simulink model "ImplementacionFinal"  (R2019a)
settings: Solver=FixedStepAuto  StartTime=0.0  StopTime=Inf  RelTol=1e-3  EnableMultiTasking=on
undefined symbols (not defined in the file): ADCIN0, ADCIN1, ADCINA0, ADCINB0, bit, ended, input, Single
libraries: c2837xDlib x6, powerlib_meascontrol x5, simulink x4, c2802xlib x3

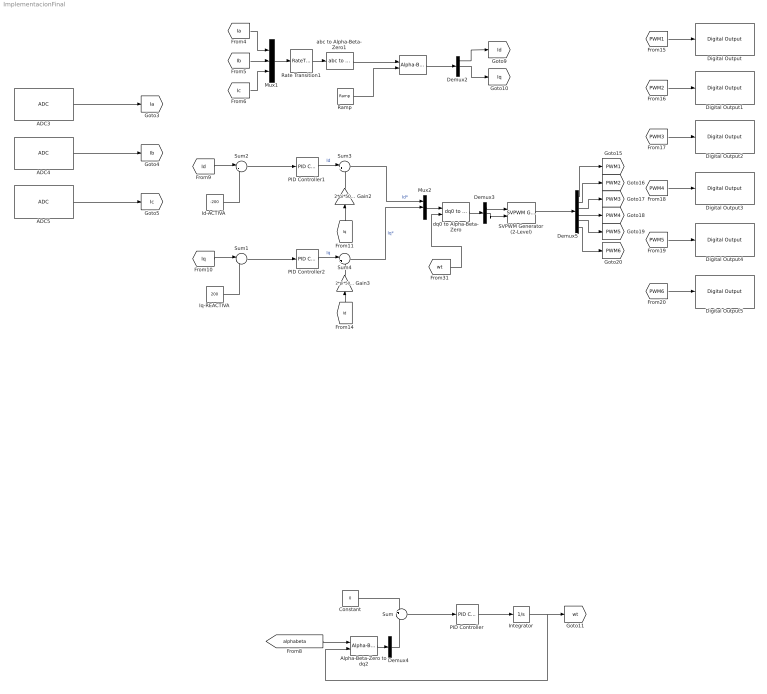
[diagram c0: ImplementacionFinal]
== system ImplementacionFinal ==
  " " : powerlib_meascontrol/Transformations/Alpha-Beta-Zero to dq0  Alignment=90 degrees behind phase A axis
  ADC3 : c2802xlib/ADC  blkParamProc=C2000_Type4  ADCModule=C  samplingMode=Single sample mode  ADCResolution=12-bit (Single-ended input)  useSOC1=SOC0  useSOC2=SOC0_SOC1  SOCAcquisitionWindow=15  SOCTriggerSource=Software  SOCInterruptTrigger=No ADCINT  Ts=0.001  dType=double  postInterrupt=off  interruptSel=ADCINT1  ADCINTContinuous=on  endma=off  chdma=1  conv1=ADCINA0  conv2=ADCINA0 and ADCINB0  conv1_Type4=ADCIN2  conv2_Type4=ADCIN0 and ADCIN1
  ADC4 : c2802xlib/ADC  blkParamProc=C2000_Type4  ADCModule=B  samplingMode=Single sample mode  ADCResolution=12-bit (Single-ended input)  useSOC1=SOC1  useSOC2=SOC0_SOC1  SOCAcquisitionWindow=15  SOCTriggerSource=Software  SOCInterruptTrigger=No ADCINT  Ts=0.001  dType=double  postInterrupt=off  interruptSel=ADCINT1  ADCINTContinuous=on  endma=off  chdma=1  conv1=ADCINA0  conv2=ADCINA0 and ADCINB0  conv1_Type4=ADCIN2  conv2_Type4=ADCIN0 and ADCIN1
  ADC5 : c2802xlib/ADC  blkParamProc=C2000_Type4  ADCModule=A  samplingMode=Single sample mode  ADCResolution=12-bit (Single-ended input)  useSOC1=SOC2  useSOC2=SOC0_SOC1  SOCAcquisitionWindow=15  SOCTriggerSource=Software  SOCInterruptTrigger=No ADCINT  Ts=0.001  dType=double  postInterrupt=off  interruptSel=ADCINT1  ADCINTContinuous=on  endma=off  chdma=1  conv1=ADCINA0  conv2=ADCINA0 and ADCINB0  conv1_Type4=ADCIN2  conv2_Type4=ADCIN0 and ADCIN1
  Alpha-Beta-Zero to dq2 : powerlib_meascontrol/Transformations/Alpha-Beta-Zero to dq0  Alignment=90 degrees behind phase A axis
  Constant : Constant  Value=0
  Demux2 : Demux  Outputs=3
  Demux3 : Demux  Outputs=3
  Demux4 : Demux  Outputs=3
  Demux5 : Demux  Outputs=6
  Digital Output : c2837xDlib/Digital Output  GPIO_Number=GPIO0~GPIO7  GPIO_Bit0=on  GPIO_BIT0_Toggle=off  GPIO_Bit1=off  GPIO_BIT1_Toggle=off  GPIO_Bit2=off  GPIO_BIT2_Toggle=off  GPIO_Bit3=off  GPIO_BIT3_Toggle=off  GPIO_Bit4=off  GPIO_BIT4_Toggle=off  GPIO_Bit5=off  GPIO_BIT5_Toggle=off  GPIO_Bit6=off  GPIO_BIT6_Toggle=off  GPIO_Bit7=off  GPIO_BIT7_Toggle=off
  Digital Output1 : c2837xDlib/Digital Output  GPIO_Number=GPIO0~GPIO7  GPIO_Bit0=off  GPIO_BIT0_Toggle=off  GPIO_Bit1=on  GPIO_BIT1_Toggle=off  GPIO_Bit2=off  GPIO_BIT2_Toggle=off  GPIO_Bit3=off  GPIO_BIT3_Toggle=off  GPIO_Bit4=off  GPIO_BIT4_Toggle=off  GPIO_Bit5=off  GPIO_BIT5_Toggle=off  GPIO_Bit6=off  GPIO_BIT6_Toggle=off  GPIO_Bit7=off  GPIO_BIT7_Toggle=off
  Digital Output2 : c2837xDlib/Digital Output  GPIO_Number=GPIO0~GPIO7  GPIO_Bit0=off  GPIO_BIT0_Toggle=off  GPIO_Bit1=off  GPIO_BIT1_Toggle=off  GPIO_Bit2=on  GPIO_BIT2_Toggle=off  GPIO_Bit3=off  GPIO_BIT3_Toggle=off  GPIO_Bit4=off  GPIO_BIT4_Toggle=off  GPIO_Bit5=off  GPIO_BIT5_Toggle=off  GPIO_Bit6=off  GPIO_BIT6_Toggle=off  GPIO_Bit7=off  GPIO_BIT7_Toggle=off
  Digital Output3 : c2837xDlib/Digital Output  GPIO_Number=GPIO0~GPIO7  GPIO_Bit0=off  GPIO_BIT0_Toggle=off  GPIO_Bit1=off  GPIO_BIT1_Toggle=off  GPIO_Bit2=off  GPIO_BIT2_Toggle=off  GPIO_Bit3=on  GPIO_BIT3_Toggle=off  GPIO_Bit4=off  GPIO_BIT4_Toggle=off  GPIO_Bit5=off  GPIO_BIT5_Toggle=off  GPIO_Bit6=off  GPIO_BIT6_Toggle=off  GPIO_Bit7=off  GPIO_BIT7_Toggle=off
  Digital Output4 : c2837xDlib/Digital Output  GPIO_Number=GPIO0~GPIO7  GPIO_Bit0=off  GPIO_BIT0_Toggle=off  GPIO_Bit1=off  GPIO_BIT1_Toggle=off  GPIO_Bit2=off  GPIO_BIT2_Toggle=off  GPIO_Bit3=off  GPIO_BIT3_Toggle=off  GPIO_Bit4=on  GPIO_BIT4_Toggle=off  GPIO_Bit5=off  GPIO_BIT5_Toggle=off  GPIO_Bit6=off  GPIO_BIT6_Toggle=off  GPIO_Bit7=off  GPIO_BIT7_Toggle=off
  Digital Output5 : c2837xDlib/Digital Output  GPIO_Number=GPIO0~GPIO7  GPIO_Bit0=off  GPIO_BIT0_Toggle=off  GPIO_Bit1=off  GPIO_BIT1_Toggle=off  GPIO_Bit2=off  GPIO_BIT2_Toggle=off  GPIO_Bit3=off  GPIO_BIT3_Toggle=off  GPIO_Bit4=off  GPIO_BIT4_Toggle=off  GPIO_Bit5=on  GPIO_BIT5_Toggle=off  GPIO_Bit6=off  GPIO_BIT6_Toggle=off  GPIO_Bit7=off  GPIO_BIT7_Toggle=off
  Gain2 : Gain  Gain=2*pi*50*1000e-6
  Gain3 : Gain  Gain=2*pi*50*1000e-6
  "Id-ACTIVA " : Constant  Value=-200
  Integrator : Integrator
  Iq-REACTIVA : Constant  Value=200
  Mux1 : Mux  Inputs=3
  Mux2 : Mux  Inputs=3
  PID Controller : simulink/Continuous/PID Controller  Controller=PI  Form=Parallel  TimeDomain=Continuous-time  SampleTime=-1  IntegratorMethod=Forward Euler  FilterMethod=Forward Euler  ControllerParametersSource=internal  P=10  I=50000  D=0  UseFilter=on  N=100  TunerSelectOption=Transfer Function Based (PID Tuner App)  InitialConditionSource=internal  InitialConditionForIntegrator=0  InitialConditionForFilter=0  DifferentiatorICPrevScaledInput=0  ExternalReset=none  TrackingMode=off  Kt=1  LimitOutput=off  UpperSaturationLimit=inf  LowerSaturationLimit=-inf  LinearizeAsGain=on  AntiWindupMode=none  Kb=1  POutMin=[]  POutMax=[]  IOutMin=[]  IOutMax=[]  DOutMin=[]  DOutMax=[]  NOutMin=[]  NOutMax=[]  SumOutMin=[]  SumOutMax=[]  SaturationOutMin=[]  SaturationOutMax=[]  PParamMin=[]  PParamMax=[]  IParamMin=[]  IParamMax=[]  DParamMin=[]  DParamMax=[]  NParamMin=[]  NParamMax=[]  KbParamMin=[]  KbParamMax=[]  KtParamMin=[]  KtParamMax=[]  KbOutMin=[]  KbOutMax=[]  KtOutMin=[]  KtOutMax=[]  IntegratorOutMin=[]  IntegratorOutMax=[]  FilterOutMin=[]  FilterOutMax=[]  SumI1OutMin=[]  SumI1OutMax=[]  SumI2OutMin=[]  SumI2OutMax=[]  SumI3OutMin=[]  SumI3OutMax=[]  SumI4OutMin=[]  SumI4OutMax=[]  SumDOutMin=[]  SumDOutMax=[]  DifferentiatorOutMin=[]  DifferentiatorOutMax=[]  FilterDiffOutCoefMin=[]  FilterDiffOutCoefMax=[]  ReciprocalOutMin=[]  ReciprocalOutMax=[]  SumDenOutMin=[]  SumDenOutMax=[]  SumNumOutMin=[]  SumNumOutMax=[]  DivideOutMin=[]  DivideOutMax=[]  IntegratorContinuousStateAttributes=''  IntegratorStateMustResolveToSignalObject=off  IntegratorRTWStateStorageClass=Auto  FilterContinuousStateAttributes=''  FilterStateMustResolveToSignalObject=off  FilterRTWStateStorageClass=Auto  ParallelPVariant=InternalParameters  IdealPVariant=Disabled  IVariant=InternalParameters  DVariant=Disabled  IntegratorVariant=Continuous  SatVariant=Disabled  AWVariant=Passthrough  PCopyVariant=Disabled  TRVariant=Disabled  FdbkBlocksVariant=Forward  IdealPFdbkVariant=Disabled  SatFdbkVariant=Disabled  DerivativeFilterVariant=Disabled  NVariant=Disabled  NCopyVariant=Disabled_SignalSpec  FilterICVariant=Disabled  IntegratorICVariant=InternalICs  ExternalResetVariant=Disabled  TRSumVariant=Passthrough  SumFdbkVariant=Disabled  SumVariant=Sum_PI
  PID Controller1 : simulink/Continuous/PID Controller  Controller=PI  Form=Parallel  TimeDomain=Continuous-time  SampleTime=-1  IntegratorMethod=Forward Euler  FilterMethod=Forward Euler  ControllerParametersSource=internal  P=5  I=5000  D=0  UseFilter=on  N=100  TunerSelectOption=Transfer Function Based (PID Tuner App)  InitialConditionSource=internal  InitialConditionForIntegrator=0  InitialConditionForFilter=0  DifferentiatorICPrevScaledInput=0  ExternalReset=none  TrackingMode=off  Kt=1  LimitOutput=off  UpperSaturationLimit=inf  LowerSaturationLimit=-inf  LinearizeAsGain=on  AntiWindupMode=none  Kb=1  POutMin=[]  POutMax=[]  IOutMin=[]  IOutMax=[]  DOutMin=[]  DOutMax=[]  NOutMin=[]  NOutMax=[]  SumOutMin=[]  SumOutMax=[]  SaturationOutMin=[]  SaturationOutMax=[]  PParamMin=[]  PParamMax=[]  IParamMin=[]  IParamMax=[]  DParamMin=[]  DParamMax=[]  NParamMin=[]  NParamMax=[]  KbParamMin=[]  KbParamMax=[]  KtParamMin=[]  KtParamMax=[]  KbOutMin=[]  KbOutMax=[]  KtOutMin=[]  KtOutMax=[]  IntegratorOutMin=[]  IntegratorOutMax=[]  FilterOutMin=[]  FilterOutMax=[]  SumI1OutMin=[]  SumI1OutMax=[]  SumI2OutMin=[]  SumI2OutMax=[]  SumI3OutMin=[]  SumI3OutMax=[]  SumI4OutMin=[]  SumI4OutMax=[]  SumDOutMin=[]  SumDOutMax=[]  DifferentiatorOutMin=[]  DifferentiatorOutMax=[]  FilterDiffOutCoefMin=[]  FilterDiffOutCoefMax=[]  ReciprocalOutMin=[]  ReciprocalOutMax=[]  SumDenOutMin=[]  SumDenOutMax=[]  SumNumOutMin=[]  SumNumOutMax=[]  DivideOutMin=[]  DivideOutMax=[]  IntegratorContinuousStateAttributes=''  IntegratorStateMustResolveToSignalObject=off  IntegratorRTWStateStorageClass=Auto  FilterContinuousStateAttributes=''  FilterStateMustResolveToSignalObject=off  FilterRTWStateStorageClass=Auto  ParallelPVariant=InternalParameters  IdealPVariant=Disabled  IVariant=InternalParameters  DVariant=Disabled  IntegratorVariant=Continuous  SatVariant=Disabled  AWVariant=Passthrough  PCopyVariant=Disabled  TRVariant=Disabled  FdbkBlocksVariant=Forward  IdealPFdbkVariant=Disabled  SatFdbkVariant=Disabled  DerivativeFilterVariant=Disabled  NVariant=Disabled  NCopyVariant=Disabled_SignalSpec  FilterICVariant=Disabled  IntegratorICVariant=InternalICs  ExternalResetVariant=Disabled  TRSumVariant=Passthrough  SumFdbkVariant=Disabled  SumVariant=Sum_PI
  PID Controller2 : simulink/Continuous/PID Controller  Controller=PI  Form=Parallel  TimeDomain=Continuous-time  SampleTime=-1  IntegratorMethod=Forward Euler  FilterMethod=Forward Euler  ControllerParametersSource=internal  P=5  I=5000  D=0  UseFilter=on  N=100  TunerSelectOption=Transfer Function Based (PID Tuner App)  InitialConditionSource=internal  InitialConditionForIntegrator=0  InitialConditionForFilter=0  DifferentiatorICPrevScaledInput=0  ExternalReset=none  TrackingMode=off  Kt=1  LimitOutput=off  UpperSaturationLimit=inf  LowerSaturationLimit=-inf  LinearizeAsGain=on  AntiWindupMode=none  Kb=1  POutMin=[]  POutMax=[]  IOutMin=[]  IOutMax=[]  DOutMin=[]  DOutMax=[]  NOutMin=[]  NOutMax=[]  SumOutMin=[]  SumOutMax=[]  SaturationOutMin=[]  SaturationOutMax=[]  PParamMin=[]  PParamMax=[]  IParamMin=[]  IParamMax=[]  DParamMin=[]  DParamMax=[]  NParamMin=[]  NParamMax=[]  KbParamMin=[]  KbParamMax=[]  KtParamMin=[]  KtParamMax=[]  KbOutMin=[]  KbOutMax=[]  KtOutMin=[]  KtOutMax=[]  IntegratorOutMin=[]  IntegratorOutMax=[]  FilterOutMin=[]  FilterOutMax=[]  SumI1OutMin=[]  SumI1OutMax=[]  SumI2OutMin=[]  SumI2OutMax=[]  SumI3OutMin=[]  SumI3OutMax=[]  SumI4OutMin=[]  SumI4OutMax=[]  SumDOutMin=[]  SumDOutMax=[]  DifferentiatorOutMin=[]  DifferentiatorOutMax=[]  FilterDiffOutCoefMin=[]  FilterDiffOutCoefMax=[]  ReciprocalOutMin=[]  ReciprocalOutMax=[]  SumDenOutMin=[]  SumDenOutMax=[]  SumNumOutMin=[]  SumNumOutMax=[]  DivideOutMin=[]  DivideOutMax=[]  IntegratorContinuousStateAttributes=''  IntegratorStateMustResolveToSignalObject=off  IntegratorRTWStateStorageClass=Auto  FilterContinuousStateAttributes=''  FilterStateMustResolveToSignalObject=off  FilterRTWStateStorageClass=Auto  ParallelPVariant=InternalParameters  IdealPVariant=Disabled  IVariant=InternalParameters  DVariant=Disabled  IntegratorVariant=Continuous  SatVariant=Disabled  AWVariant=Passthrough  PCopyVariant=Disabled  TRVariant=Disabled  FdbkBlocksVariant=Forward  IdealPFdbkVariant=Disabled  SatFdbkVariant=Disabled  DerivativeFilterVariant=Disabled  NVariant=Disabled  NCopyVariant=Disabled_SignalSpec  FilterICVariant=Disabled  IntegratorICVariant=InternalICs  ExternalResetVariant=Disabled  TRSumVariant=Passthrough  SumFdbkVariant=Disabled  SumVariant=Sum_PI
  Ramp : simulink/Sources/Ramp  slope=315  start=0  InitialOutput=-2.6
  Rate Transition1 : RateTransition
  SVPWM Generator (2-Level) : powerlib_meascontrol/Pulse & Signal Generators/SVPWM Generator (2-Level)  InputType=alpha-beta components  SwitchingPattern=Pattern #1  Fc=2000  ParUref=[0.8 -30 50]  Ts=0
  Sum : Sum  Inputs=+-
  Sum1 : Sum  Inputs=|-+
  Sum2 : Sum  Inputs=|-+
  Sum3 : Sum  Inputs=|++
  Sum4 : Sum  Inputs=|+-
  abc to Alpha-Beta-Zero1 : powerlib_meascontrol/Transformations/abc to Alpha-Beta-Zero
  dq0 to Alpha-Beta-Zero : powerlib_meascontrol/Transformations/dq0 to Alpha-Beta-Zero  Alignment=90 degrees behind phase A axis
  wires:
  Sum4/1 -> Mux2/2  "Iq*"
  [Id] -> Gain3/1
  Sum1/1 -> PID Controller2/1
  PID Controller2/1 -> Sum4/1  "Iq"
  Iq-REACTIVA/1 -> Sum1/2
  [Id] -> Sum2/1
  Integrator/1 -> Alpha-Beta-Zero to dq2/2, [wt]
  PID Controller/1 -> Integrator/1
  " "/1 -> Demux2/1
  [Ib] -> Mux1/2
  Demux2/1 -> [Id]
  [Ic] -> Mux1/3
  Sum2/1 -> PID Controller1/1
  [Ia] -> Mux1/1
  Demux2/2 -> [Iq]
  [Iq] -> Gain2/1
  Gain3/1 -> Sum4/2
  PID Controller1/1 -> Sum3/1  "Id"
  [alphabeta] -> Alpha-Beta-Zero to dq2/1
  Constant/1 -> Sum/1
  Sum/1 -> PID Controller/1
  Gain2/1 -> Sum3/2
  "Id-ACTIVA "/1 -> Sum2/2
  [Iq] -> Sum1/1
  Demux5/5 -> [PWM5]
  Demux5/1 -> [PWM1]
  Demux5/4 -> [PWM4]
  Demux5/6 -> [PWM6]
  Demux5/3 -> [PWM3]
  Demux5/2 -> [PWM2]
  Alpha-Beta-Zero to dq2/1 -> Demux4/1
  Mux2/1 -> dq0 to Alpha-Beta-Zero/1
  [wt] -> dq0 to Alpha-Beta-Zero/2
  SVPWM Generator (2-Level)/1 -> Demux5/1
  dq0 to Alpha-Beta-Zero/1 -> Demux3/1
  Demux3/1 -> SVPWM Generator (2-Level)/1
  Demux3/2 -> SVPWM Generator (2-Level)/2
  ADC5/1 -> [Ic]
  ADC4/1 -> [Ib]
  ADC3/1 -> [Ia]
  [PWM1] -> Digital Output/1
  [PWM2] -> Digital Output1/1
  [PWM3] -> Digital Output2/1
  [PWM4] -> Digital Output3/1
  [PWM5] -> Digital Output4/1
  [PWM6] -> Digital Output5/1
  Mux1/1 -> Rate Transition1/1
  Rate Transition1/1 -> abc to Alpha-Beta-Zero1/1
  Demux4/2 -> Sum/2
  abc to Alpha-Beta-Zero1/1 -> " "/1
  Ramp/1 -> " "/2
  Sum3/1 -> Mux2/1  "Id*"
